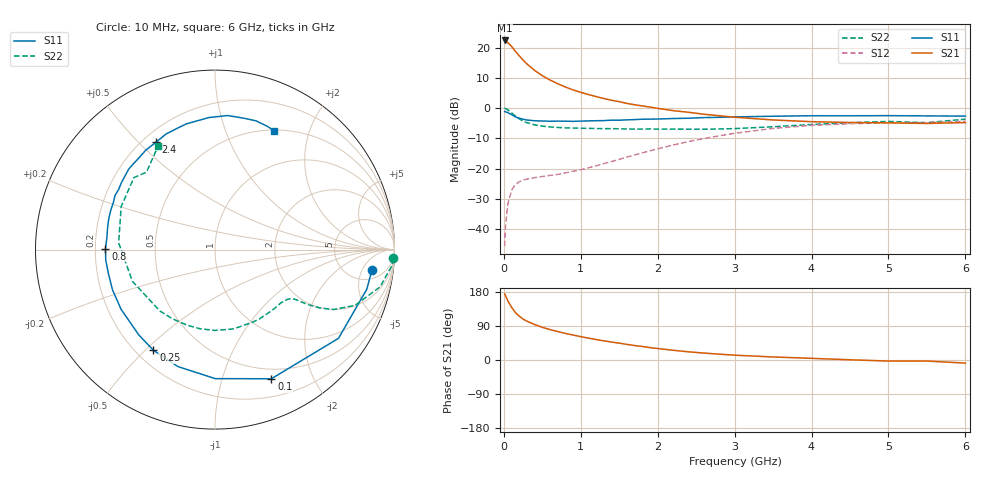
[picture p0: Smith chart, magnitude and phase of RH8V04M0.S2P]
! SIEMENS Small Signal Semiconductors
! BFR106
! Si NPN RF Bipolar Junction Transistor in SOT23
! VCE = 8 V  IC = 4 mA
! Common Emitter S-Parameters:  August  1996
# GHz  S  MA  R  50
!  f  S11  S21  S12  S22
! GHz  MAG  ANG  MAG  ANG  MAG  ANG  MAG  ANG
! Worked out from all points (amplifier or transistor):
!   36 points, 10 MHz to 6 GHz, reference 50 ohm
!   highest |S21| = 22.4 dB at 10 MHz (marker M1)
!   |S21| within 3 dB of that: start of sweep to 132 MHz
!   unconditionally stable (mu >= 1): 672.9 MHz to 1.811 GHz; 4.775 GHz to end of sweep
!   at 250 MHz: K = 0.44, MSG = 19.8 dB, |S12| = -23.8 dB
!   at 1.4 GHz: K = 1.14, MAG = 7.8 dB, |S12| = -17.7 dB
!   at 6 GHz: K = 1.02, MAG = -1.1 dB, |S12| = -4.3 dB
!   S11 on the Smith chart (normalised r, x): 10 MHz: 8, -8; 100 MHz: 0.39, -1.46; 250 MHz: 0.27, -0.53; 800 MHz: 0.24, +0.00; 2.4 GHz: 0.25, +0.56; 6 GHz: 0.51, +1.49
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0.01  0.8815 -7.4  13.23 174.6  0.0052 88.4  0.9952 -2.8
0.02  0.8743 -14.6  13.06 170.7  0.0107 83.9  0.9882 -5.4
0.05  0.8472 -35.7  12.23 156.9  0.0252 71.2  0.9431 -12.7
0.1  0.7852 -66.4  10.57 139.4  0.0437 58.2  0.8399 -21.7
0.15  0.719 -89.9  8.751 125.1  0.0545 48.4  0.7406 -26.8
0.2  0.6836 -107.6  7.384 115.9  0.0605 42.8  0.669 -29.1
0.25  0.6574 -121.5  6.264 107.9  0.0649 39.3  0.6117 -30.4
0.3  0.6371 -131.9  5.397 102.4  0.0669 38.3  0.5759 -31.0
0.4  0.62 -147.6  4.226 93.6  0.0709 37.5  0.53 -31.7
0.5  0.6135 -158.5  3.448 86.2  0.0739 38.6  0.5046 -32.6
0.6  0.6087 -167.4  2.931 80.3  0.0772 41.2  0.4897 -34.4
0.8  0.6101 179.5  2.242 70.2  0.0851 47.8  0.4724 -38.7
1.1  0.6166 163.6  1.684 57.7  0.1031 57.3  0.464 -47.3
1.3  0.6238 155.2  1.446 50.5  0.1211 62.1  0.459 -53.7
1.6  0.6417 144.2  1.199 41.2  0.1551 66.4  0.454 -64.7
2.2  0.6752 124.8  0.912 25.7  0.2458 65.5  0.4502 -90.3
2.4  0.6825 118.8  0.856 21.6  0.2801 63.1  0.4488 -100.7
3.5  0.7363 92.7  0.639 8.0  0.4627 42.6  0.4929 -159.0
4.5  0.7494 77.9  0.58 0.6  0.5535 21.4  0.5749 155.4
5  0.7529 72.3  0.572 -2.8  0.5736 12.7  0.6041 138.4
5.5  0.7459 66.9  0.559 -2.8  0.5766 8.3  0.5761 131.5
6  0.7397 63.5  0.578 -8.2  0.609 -0.1  0.6587 118.7
